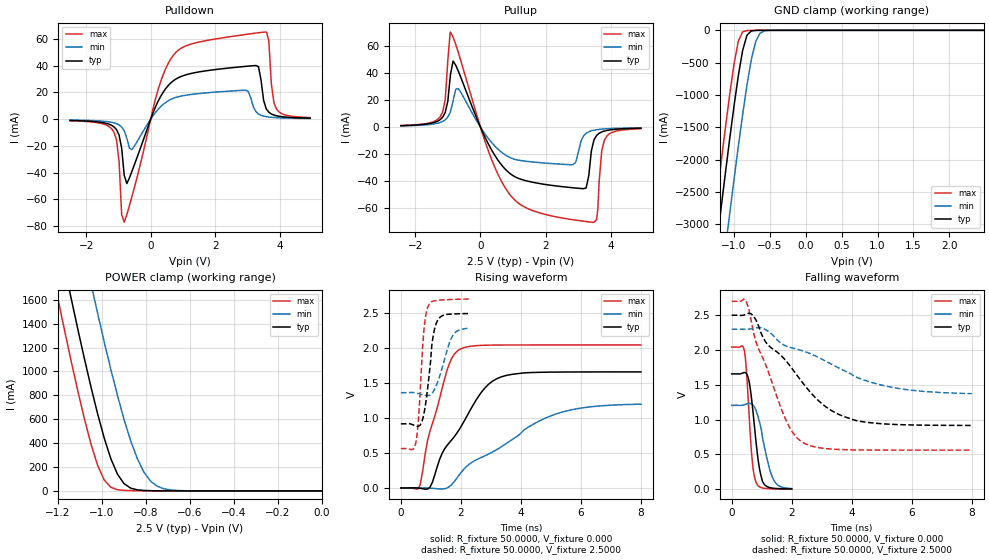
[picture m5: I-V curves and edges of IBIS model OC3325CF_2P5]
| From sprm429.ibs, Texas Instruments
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|   Model OC3325CF_2P5
[Model]   OC3325CF_2P5
Model_type   3-state
Polarity   Non-Inverting
Enable   Active-Low
Vmeas =   1.2500V
Cref =  15.0000pF
Rref = 100.0000M
Vref =  0.000V
C_comp   3.2400pF   3.2484pF   3.2323pF
[Temperature Range]   25.0000   0.1250k   -40.0000
[Pullup Reference]   2.5000V   2.3000V   2.7000V
[Pulldown Reference]   0.000V   0.000V   0.000V
[POWER Clamp Reference]   2.5000V   2.3000V   2.7000V
[GND Clamp Reference]   0.000V   0.000V   0.000V
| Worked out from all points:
|   slope of the pulldown table from 0 to 0.375 V, typ, clamps not added: 19 ohm
|   slope of the pullup table from 0 to 0.375 V, typ, clamps not added: 20.5 ohm
|   GND clamp passes 1 mA (typ) near -0.69 V on its own axis
|   POWER clamp passes 1 mA (typ) near -0.74 V on its own axis
|   rising waveform, R_fixture 50.0000, V_fixture 0.000: 20-80 % time 1.38ns typ, 2.58ns min, 725ps max; typ from 0 V to 1.66 V
|   rising waveform, R_fixture 50.0000, V_fixture 2.5000: 20-80 % time 244ps typ, 391ps min, 184ps max; typ from 0.916 V to 2.49 V
|   falling waveform, R_fixture 50.0000, V_fixture 0.000: 20-80 % time 257ps typ, 367ps min, 183ps max; typ from 1.66 V to 0.005 V
|   falling waveform, R_fixture 50.0000, V_fixture 2.5000: 20-80 % time 1.95ns typ, 2.89ns min, 1.1ns max; typ from 2.5 V to 0.917 V
[Pulldown]
| voltage   I(typ)   I(min)   I(max)
-2.5V     -991uA     -679uA     -1.209mA
-1.14V    -5.745mA   -2.795mA   -9.669mA
-980mV    -11.89mA   -4.32mA    -31.77mA
-820mV    -42.11mA   -8.654mA   -77.13mA
-580mV    -38.96mA   -22.79mA   -57.9mA
300mV     16.63mA    9.087mA    27.43mA
940mV     31.88mA    17.23mA    53.01mA
2.94V     39.47mA    21.56mA    63.32mA
3.26V     40.09mA    5.59mA     64.38mA
3.6V      7.132mA    1.775mA    64.91mA
3.9V      2.485mA    1.067mA    7.487mA
4.94V     734uA      441uA      1.128mA
[Pullup]
| voltage   I(typ)   I(min)   I(max)
-2.44V    1.068mA    874uA      1.183mA
-1.24V    5.419mA    3.418mA    7.463mA
-1.08V    10.87mA    5.415mA    20.27mA
-920mV    38.79mA    11.43mA    70.36mA
-680mV    41.52mA    28.54mA    55.4mA
920mV     -34.64mA   -22.68mA   -50.49mA
2.84V     -44.93mA   -27.74mA   -68.59mA
3.24V     -45.04mA   -4.57mA    -69.93mA
3.48V     -9.548mA   -2.283mA   -70.4mA
3.56V     -6.214mA   -1.945mA   -68.62mA
3.8V      -2.9mA     -1.339mA   -9.639mA
4.92V     -795uA     -536uA     -1.172mA
[GND_clamp]
| voltage   I(typ)   I(min)   I(max)
-2.5V     -15.5A     -16.63A    -14.84A
-1.3V     -3.859A    -5.036A    -3.154A
-1.24V    -3.299A    -4.476A    -2.593A
-1.18V    -2.747A    -3.922A    -2.042A
-1.12V    -2.203A    -3.373A    -1.504A
-1.06V    -1.674A    -2.833A    -988.8mA
-940mV    -699.3mA   -1.791A    -163mA
-880mV    -309.8mA   -1.301A    -22.68mA
-820mV    -75.99mA   -847.7mA   -4.032mA
-700mV    -1.225mA   -180.1mA   -233.9uA
-580mV    -25.34uA   -9.081mA   -6.925uA
2.48V     157.2pA    34.41nA    144.3pA
[POWER_clamp]
| voltage   I(typ)   I(min)   I(max)
-2.49V    14.54A     15.38A     14.07A
-1.2V     2.135A     3.04A      1.604A
-1.14V    1.608A     2.506A     1.083A
-1.05V    867.5mA    1.733A     390.3mA
-1.02V    644.3mA    1.486A     213.7mA
-990mV    441.9mA    1.246A     91.12mA
-930mV    140.4mA    799.1mA    10.23mA
-900mV    61.07mA    598.5mA    4.539mA
-840mV    8.987mA    271.4mA    1.894mA
-780mV    1.955mA    82.94mA    922.8uA
-660mV    264.9uA    3.855mA    99.56uA
0V        159.5pA    1.158nA    167.9pA
[Ramp]
| variable   typ   min   max
dV/dt_r   0.9945/1.3702n   0.7180/2.6322n   1.2254/0.7177n
dV/dt_f   0.9497/1.9336n   0.5557/2.9406n   1.2825/1.0851n
R_load = 50.0000
[Rising Waveform]
R_fixture = 50.0000
V_fixture = 0.000
V_fixture_min = 0.000
V_fixture_max = 0.000
| time   V(typ)   V(min)   V(max)
0s        1.101nV    5.323nV    786.3pV
646.5ps   -4.403mV   993.2uV    47.76mV
969.7ps   10.51mV    -2.15mV    810.8mV
1.293ns   409.8mV    -13.85mV   1.28V
1.535ns   605.5mV    -663.5uV   1.676V
1.939ns   831.2mV    183.7mV    1.973V
2.748ns   1.401V     448.9mV    2.037V
3.394ns   1.593V     600.7mV    2.041V
5.333ns   1.656V     1.078V     2.042V
8ns       1.657V     1.197V     2.042V
[Rising Waveform]
R_fixture = 50.0000
V_fixture = 2.5000
V_fixture_min = 2.3000
V_fixture_max = 2.7000
| time   V(typ)   V(min)   V(max)
0s        916.3mV    1.361V     562.5mV
383.8ps   905.2mV    1.363V     550.3mV
505.1ps   884mV      1.356V     658.9mV
585.9ps   881.3mV    1.348V     974.6mV
767.7ps   1.058V     1.327V     2.249V
909.1ps   1.485V     1.32V      2.594V
1.051ns   2.099V     1.361V     2.665V
1.232ns   2.399V     1.521V     2.68V
1.717ns   2.483V     2.166V     2.692V
2.263ns   2.491V     2.284V     2.698V
[Falling Waveform]
R_fixture = 50.0000
V_fixture = 0.000
V_fixture_min = 0.000
V_fixture_max = 0.000
| time   V(typ)   V(min)   V(max)
0s        1.658V     1.206V     2.042V
424.2ps   1.677V     1.216V     1.987V
484.8ps   1.666V     1.224V     1.74V
545.5ps   1.609V     1.231V     1.329V
666.7ps   1.283V     1.227V     495.6mV
808.1ps   693.2mV    1.134V     104.9mV
929.3ps   289.9mV    962.2mV    35.13mV
1.071ns   79.29mV    649.9mV    15.53mV
1.434ns   13.21mV    108.7mV    5.417mV
2ns       5.144mV    10.7mV     1.868mV
[Falling Waveform]
R_fixture = 50.0000
V_fixture = 2.5000
V_fixture_min = 2.3000
V_fixture_max = 2.7000
| time   V(typ)   V(min)   V(max)
0s        2.5V       2.3V       2.7V
484.8ps   2.516V     2.298V     2.696V
808.1ps   2.433V     2.319V     2.118V
1.131ns   2.116V     2.293V     1.789V
1.697ns   1.899V     2.083V     1.107V
2.343ns   1.542V     1.992V     680mV
3.152ns   1.181V     1.836V     584.3mV
4.121ns   989.3mV    1.616V     565.3mV
5.657ns   928mV      1.442V     562.6mV
8ns       917.1mV    1.374V     562.5mV
